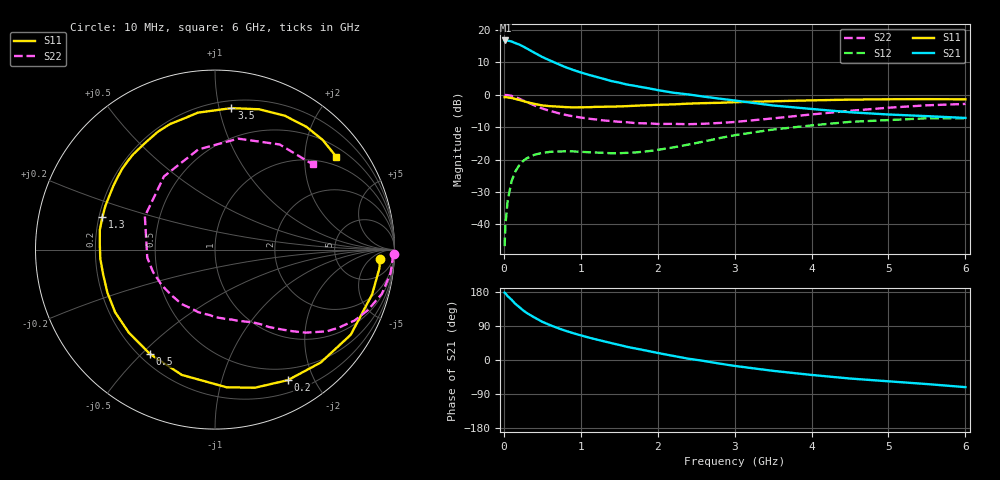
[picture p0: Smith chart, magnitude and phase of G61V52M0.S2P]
! SIEMENS Small Signal Semiconductors
! BFG193
! Si NPN RF Bipolar Junction Transistor in SOT223
! VCE = 1.5 V  IC = 2 mA
! Common Emitter S-Parameters:  August  1996
# GHz  S  MA  R  50
!  f  S11  S21  S12  S22
! GHz  MAG  ANG  MAG  ANG  MAG  ANG  MAG  ANG
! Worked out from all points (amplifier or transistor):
!   36 points, 10 MHz to 6 GHz, reference 50 ohm
!   highest |S21| = 16.8 dB at 20 MHz (marker M1)
!   |S21| within 3 dB of that: start of sweep to 337.8 MHz
!   unconditionally stable (mu >= 1): 1.359 GHz to 2.828 GHz
!   at 250 MHz: K = 0.18, MSG = 17.7 dB, |S12| = -20.4 dB
!   at 1.4 GHz: K = 1.04, MAG = 10.0 dB, |S12| = -18.1 dB
!   at 6 GHz: K = 0.99, MSG = 0.1 dB, |S12| = -7.3 dB
!   S11 on the Smith chart (normalised r, x): 10 MHz: 17, -11; 200 MHz: 0.35, -1.65; 500 MHz: 0.24, -0.53; 1.3 GHz: 0.21, +0.13; 3.5 GHz: 0.26, +1.09; 6 GHz: 0.74, +2.77
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0.01  0.9191 -3.1  6.886 177.7  0.0046 91.8  0.9954 -1.5
0.02  0.9221 -6.4  6.896 176.4  0.0096 86.0  0.9911 -3.0
0.05  0.9103 -15.9  6.849 168.3  0.0233 80.4  0.987 -7.6
0.1  0.8928 -32.1  6.657 159.2  0.0461 72.3  0.9619 -14.8
0.15  0.8619 -46.9  6.269 148.1  0.0656 63.3  0.9168 -21.5
0.2  0.8329 -60.8  5.974 139.7  0.0816 57.1  0.8727 -26.9
0.25  0.8011 -73.9  5.582 131.1  0.0952 50.1  0.8163 -32.1
0.3  0.7698 -85.2  5.168 123.9  0.1049 45.0  0.7714 -36.2
0.4  0.7223 -104.8  4.445 111.9  0.119 35.9  0.6835 -42.6
0.5  0.6852 -121.9  3.83 100.8  0.1265 29.0  0.6138 -47.5
0.6  0.667 -136.0  3.383 92.2  0.1315 24.3  0.5636 -51.5
0.7  0.6569 -147.9  3.004 84.3  0.1329 20.5  0.5239 -55.3
0.9  0.6385 -167.2  2.422 70.9  0.1336 15.4  0.4651 -61.3
1.1  0.6427 177.2  2.038 59.5  0.1298 13.3  0.4284 -68.8
1.3  0.6532 164.0  1.759 49.4  0.1272 13.3  0.4015 -76.2
1.6  0.668 148.0  1.439 34.8  0.1269 16.3  0.377 -89.7
2.2  0.7103 123.3  1.078 10.9  0.1538 23.9  0.3558 -121.5
2.8  0.7512 103.0  0.872 -9.3  0.2138 22.0  0.367 -160.1
3.5  0.7935 83.4  0.684 -28.6  0.291 8.1  0.4325 154.6
4.5  0.8413 62.4  0.537 -48.9  0.3819 -14.7  0.5655 99.5
5.5  0.8564 45.5  0.468 -63.5  0.4337 -41.5  0.6877 58.4
6  0.851 37.5  0.439 -71.6  0.4335 -55.9  0.7227 41.1
